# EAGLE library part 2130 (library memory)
MEMORY
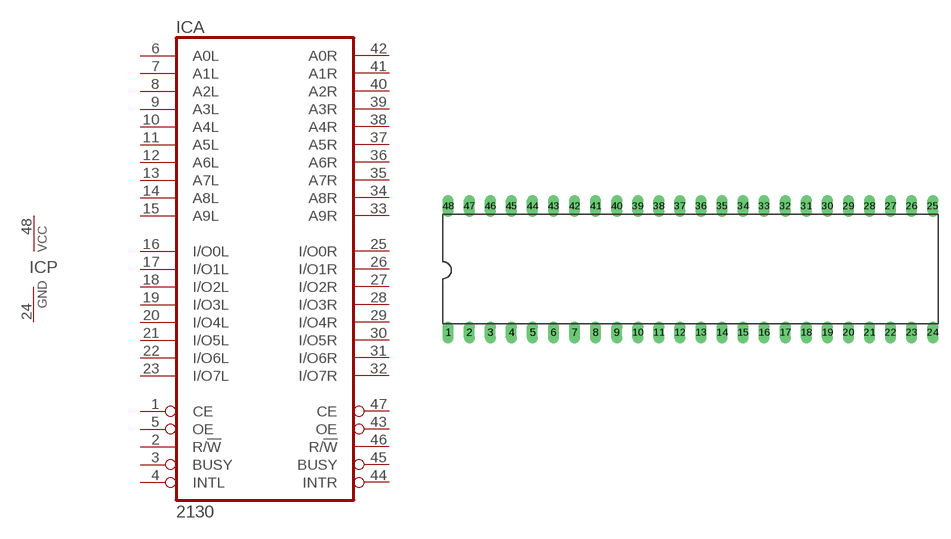
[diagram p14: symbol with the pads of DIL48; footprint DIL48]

Designator prefix IC; gates A=2130 P=PWRN

## 2130  [DIL48]
1  A:CE  in
2  A:R/!W  in
3  A:BUSY  out
4  A:INTL  out
5  A:OE  in
6  A:A0L  in
7  A:A1L  in
8  A:A2L  in
9  A:A3L  in
10  A:A4L  in
11  A:A5L  in
12  A:A6L  in
13  A:A7L  in
14  A:A8L  in
15  A:A9L  in
16  A:I/O0L
17  A:I/O1L
18  A:I/O2L
19  A:I/O3L
20  A:I/O4L
21  A:I/O5L
22  A:I/O6L
23  A:I/O7L
24  P:GND  pwr
25  A:I/O0R
26  A:I/O1R
27  A:I/O2R
28  A:I/O3R
29  A:I/O4R
30  A:I/O5R
31  A:I/O6R
32  A:I/O7R
33  A:A9R  in
34  A:A8R  in
35  A:A7R  in
36  A:A6R  in
37  A:A5R  in
38  A:A4R  in
39  A:A3R  in
40  A:A2R  in
41  A:A1R  in
42  A:A0R  in
43  A:OE  in
44  A:INTR  out
45  A:BUSY  out
46  A:R/!W  in
47  A:CE  in
48  P:VCC  pwr

## Footprint DIL48 (pad centres in mm)
Dual In Line Package
drill 0.813 long: 1 -29.21,-7.62; 2 -26.67,-7.62; 3 -24.13,-7.62; 4 -21.59,-7.62; 5 -19.05,-7.62; 6 -16.51,-7.62; 7 -13.97,-7.62; 8 -11.43,-7.62; 9 -8.89,-7.62; 10 -6.35,-7.62; 11 -3.81,-7.62; 12 -1.27,-7.62; 13 1.27,-7.62; 14 3.81,-7.62; 15 6.35,-7.62; 16 8.89,-7.62; 17 11.43,-7.62; 18 13.97,-7.62; 19 16.51,-7.62; 20 19.05,-7.62; 21 21.59,-7.62; 22 24.13,-7.62; 23 26.67,-7.62; 24 29.21,-7.62; 25 29.21,7.62; 26 26.67,7.62; 27 24.13,7.62; 28 21.59,7.62; 29 19.05,7.62; 30 16.51,7.62; 31 13.97,7.62; 32 11.43,7.62; 33 8.89,7.62; 34 6.35,7.62; 35 3.81,7.62; 36 1.27,7.62; 37 -1.27,7.62; 38 -3.81,7.62; 39 -6.35,7.62; 40 -8.89,7.62; 41 -11.43,7.62; 42 -13.97,7.62; 43 -16.51,7.62; 44 -19.05,7.62; 45 -21.59,7.62; 46 -24.13,7.62; 47 -26.67,7.62; 48 -29.21,7.62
